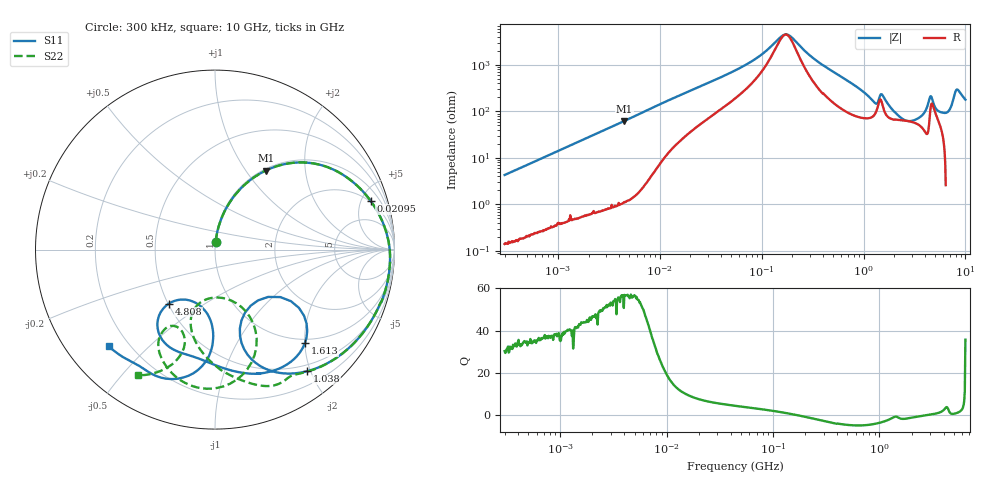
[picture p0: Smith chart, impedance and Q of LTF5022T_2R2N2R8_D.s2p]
! S-Parameter Data Generated by TDK Corporation
! Copyright(C) 2020 TDK Corporation.
! All Rights Reserved.
! TDK P/N: LTF5022T-2R2N2R8-D (Inductor)
! Property: L=2.2uH at 100kHz
! Size(LxWxT): 6.5x5x2.2mm
! Model Type: s2p (Touchstone File Format Version 1.0)
! Frequency: DC=Yes Start=0.3MHz Stop=10000MHz 802points Log-sweep
! Model Generated on Apr. 23, 2020
! Port Assignments:
!  1 ---@@@--- 2
! Applicable Conditions:
!  Temperature = 25 degC
!  DC Bias Current = 0 A
!  Small Signal Operation
! Terms and conditions regarding TDK Simulation Models
! (1)This simulation model is being provided solely for informational purposes. Please refer to the specifications of the products in terms of detailed characteristics of such products.
! (2)In no event shall TDK Corporation of any of its subsidiaries be liable for any loss or damage arising, directly or indirectly,
!  From any information contained in this simulation model, including, but not limited to loss or damages arising from any inaccuracies, omissions or errors in connection with such information.
! (3)Any and all copyrights on this simulation model are owned by TDK Corporation.
!  Duplication or redistribution of this simulation model without prior written permission from TDK Corporation is prohibited.
! (4)This simulation model is subject to any modification or change without any prior notice.
! (5)Neither TDK Corporation nor any of its subsidiaries shall make any warranty, express or implied,
!  Including but not limited to the correctness, implied warranties of merchantability and fitness for a particular purpose with respect to this simulation models.
! (6)The use of this simulation model shall be deemed to have consented to the terms and conditions hereof.
# Hz S MA R 50
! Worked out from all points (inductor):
!   801 points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, 300 kHz to 10 GHz, reference 50 ohm
!   read as one part in series: L = 2.26 uH near 318.3 kHz
!   highest Q = 56.6 at 4.487 MHz (marker M1), where L = 2.21 uH
!   self-resonance near 172.1 MHz
!   S11 on the Smith chart (normalised r, x): 300 kHz: 1.00, +0.09; 20.95 MHz: 1.90, +5.93; 1.038 GHz: 0.40, -1.95; 1.613 GHz: 0.91, -2.00; 4.808 GHz: 0.50, -0.36; 10 GHz: 0.13, -0.38
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300000  0.04294 85.8  0.9976 -2.4  0.9977 -2.5  0.04282 85.5
1713600  0.2299 75.3  0.968 -13.3  0.9679 -13.3  0.2299 75.4
4487199  0.5231 57.3  0.8428 -31.7  0.8428 -31.7  0.5231 57.3
9671944  0.789 34.9  0.5772 -52.3  0.5772 -52.3  0.7891 34.9
2.094725e7  0.9085 17.4  0.3129 -64.8  0.313 -64.8  0.9084 17.4
5.477226e7  0.9605 5.4  0.1274 -70.1  0.1274 -70.1  0.9604 5.4
1.69821e8  0.978 -5.1  0.02183 -8.4  0.02182 -8.4  0.9779 -5.2
3.126428e8  0.9759 -13.2  0.06624 58.0  0.06623 57.9  0.976 -13.2
6.573376e8  0.9419 -30.8  0.1787 48.2  0.1788 48.2  0.9441 -30.1
1.038183e9  0.8503 -52.8  0.2924 25.0  0.2933 25.2  0.8791 -47.9
1.339606e9  0.5019 -73.9  0.3218 -5.8  0.3276 -5.7  0.8214 -59.4
1.459486e9  0.4499 -36.0  0.2352 -5.5  0.2407 -6.9  0.8278 -65.1
1.613252e9  0.7233 -46.2  0.3008 5.7  0.2984 4.6  0.7821 -73.7
1.767019e9  0.755 -59.1  0.3589 -3.0  0.3557 -3.6  0.7302 -80.0
2.720446e9  0.6467 -89.2  0.4286 -53.9  0.4257 -54.0  0.4738 -105.9
3.766866e9  0.6053 -108.2  0.3459 -106.1  0.3431 -106.0  0.2672 -90.3
4.34106e9  0.5587 -124.3  0.1782 -129.8  0.1773 -129.2  0.5053 -63.5
4.807583e9  0.3958 -130.5  0.1673 -89.8  0.1683 -90.3  0.7518 -83.6
5.607117e9  0.332 -102.2  0.2831 -119.3  0.2788 -119.7  0.7374 -107.8
6.899057e9  0.5406 -91.7  0.2248 -177.7  0.2159 -176.0  0.5764 -122.3
8.211115e9  0.769 -110.7  0.08411 167.0  0.0911 170.6  0.5277 -108.6
1e10  0.7993 -137.7  0.08496 155.5  0.08508 156.4  0.8228 -121.6
